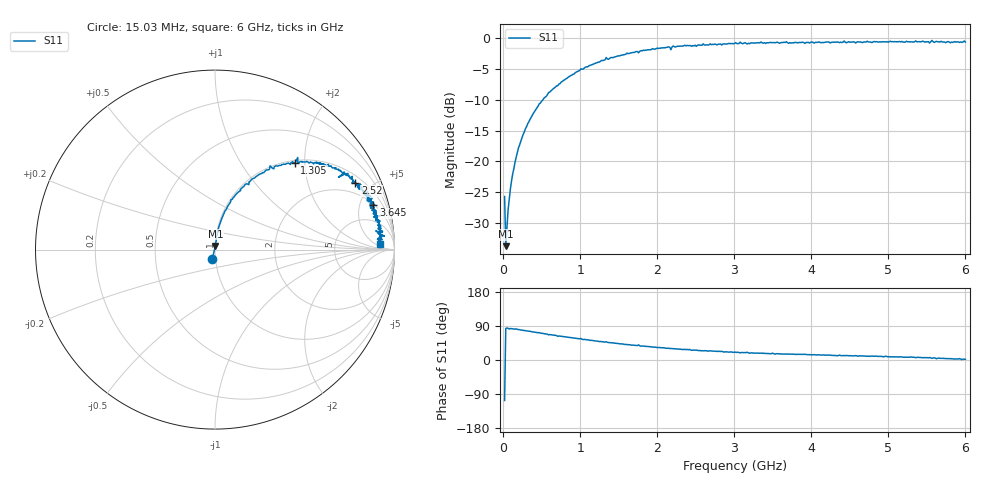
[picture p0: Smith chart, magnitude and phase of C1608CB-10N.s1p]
!	Network	Analyzer	HP8753E.07.74:	Oct	30	2002	Serial	No.	JP38451487
!	Hewlett-Packard
!	7	Sep	2009	9:34:10
!	Frequency	S11
#	HZ	S	RI	R	50
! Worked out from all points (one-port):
!   400 points, 15.03 MHz to 6 GHz, reference 50 ohm
!   lowest |S11| = -33.7 dB at 30.03 MHz (marker M1), VSWR 1.04, Z = 50.2 + j2.07 ohm
!   |S11| at or under -10 dB: start of sweep to 514.9 MHz
!   S11 on the Smith chart (normalised r, x): 15.03 MHz: 0.97, -0.10; 1.305 GHz: 1.05, +1.78; 2.52 GHz: 1.35, +4.01; 3.645 GHz: 2.11, +6.60; 6 GHz: 21, +8
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1.502992e7  -0.0151 -0.0499
3.002985e7  0.00247 0.0206
6.00297e7  0.00453 0.0403
9.002955e7  0.00729 0.0596
1.95029e8  0.0214 0.127
3.150284e8  0.047 0.196
4.650277e8  0.0891 0.278
7.650262e8  0.205 0.392
1.005025e9  0.307 0.467
1.305023e9  0.444 0.484
1.335023e9  0.461 0.513
1.515022e9  0.524 0.482
1.725021e9  0.605 0.477
1.755021e9  0.577 0.483
1.785021e9  0.628 0.466
1.93502e9  0.674 0.456
2.145019e9  0.722 0.431
2.175019e9  0.688 0.403
2.205019e9  0.741 0.424
2.265019e9  0.743 0.416
2.520017e9  0.782 0.371
3.015015e9  0.851 0.32
3.195014e9  0.849 0.271
3.645012e9  0.883 0.248
3.765011e9  0.871 0.241
4.515007e9  0.9 0.181
5.265004e9  0.917 0.119
6e9  0.919 0.0298
